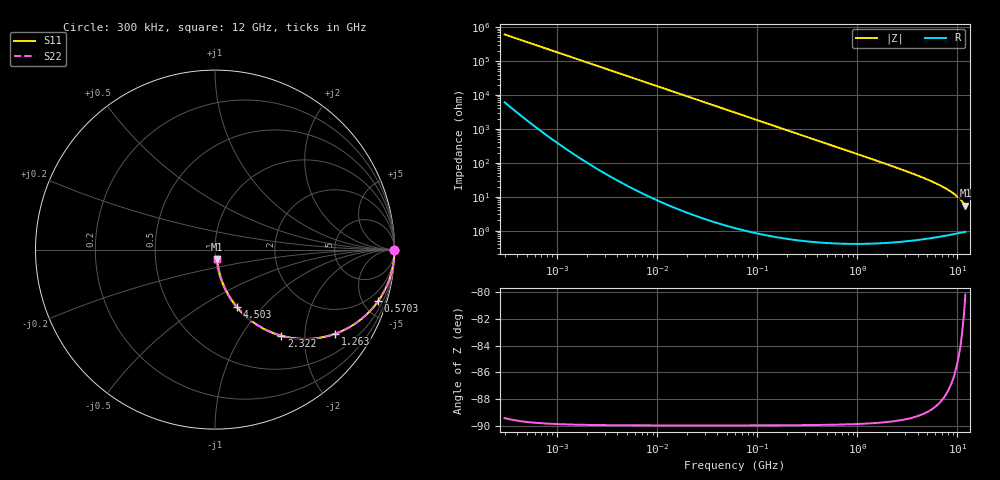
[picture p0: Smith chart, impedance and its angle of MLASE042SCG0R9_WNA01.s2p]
! MLASE042SCG0R9_WNA01  S-PARAMETER MODEL  ( General Type )
! Model Generated by TAIYO YUDEN Corporation (http://www.ty-top.com)
! Version 1.0
! TAIYO YUDEN Control No. 130801
! Copyright(c) 2013 TAIYO YUDEN CO.,LTD. All Rights Reserved.
! Product Description (link to TY-COMPAS)
! https://ds.yuden.co.jp/TYCOMPAS/or/detail?pn=MLASE042SCG0R9AWNA01&u=M
! Products Name : Multilayer Ceramic Capacitors
! Characteristics :
!  Capacitance : 0.9 pF , Rated Voltage : 16V , TCC : CG / C0G
!  Case Size : 0.4 x 0.2 / 0.016 x 0.008 [mm/inch] , Thickness : 0.2 / 0.008 [mm/inch]
!  (Conditions: Temperature = 25 degC , DC Bias Current/Voltage = 0A / 0V)
! External Node Assignments :
!  1  o---| |---o  2
! GND o---------o GND
! Frequency Range : 0.3MHz  -  12000MHz  [ 401 STEP ]
# MHz S RI R 50
! Freq[MHz].  S11 Real  S11 Imag  S21 Real  S21 Imag  S12 Real  S12 Imag  S22 Real  S22 Imag
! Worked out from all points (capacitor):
!   401 points, 300 kHz to 12 GHz, reference 50 ohm
!   read as one part in series: C = 876 fF near 316.3 kHz
!   lowest |Z| = 5.43 ohm at 12 GHz (marker M1)
!   S11 on the Smith chart (normalised r, x): 300 kHz: open; 570.3 MHz: 1.01, -6.36; 1.263 GHz: 1.01, -2.86; 2.322 GHz: 1.01, -1.53; 4.503 GHz: 1.01, -0.73; 12 GHz: 1.02, -0.11
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0.3  1 -0.000165  1.68e-06 0.000165  1.68e-06 0.000165  1 -0.000165
1.769972  1 -0.000974  2.14e-06 0.000974  2.14e-06 0.000974  1 -0.000974
10.44266  1 -0.00575  3.55e-05 0.00575  3.55e-05 0.00575  1 -0.00575
60  0.9989 -0.033  0.0011 0.033  0.0011 0.033  0.9989 -0.033
164.1901  0.9918 -0.0897  0.00815 0.0897  0.00815 0.0897  0.9918 -0.0897
244.3004  0.9821 -0.1321  0.0179 0.1321  0.0179 0.1321  0.9821 -0.1321
353.9943  0.9632 -0.1878  0.0368 0.1878  0.0368 0.1878  0.9632 -0.1878
570.2811  0.9097 -0.2859  0.0903 0.2859  0.0903 0.2859  0.9097 -0.2859
848.5281  0.8195 -0.3837  0.1805 0.3837  0.1805 0.3837  0.8195 -0.3837
1021.415  0.7576 -0.4274  0.2424 0.4274  0.2424 0.4274  0.7576 -0.4274
1262.535  0.6707 -0.4685  0.3293 0.4685  0.3293 0.4685  0.6707 -0.4685
1645.489  0.5431 -0.4962  0.4569 0.4962  0.4569 0.4962  0.5431 -0.4962
2088.533  0.4214 -0.4912  0.5786 0.4912  0.5786 0.4912  0.4214 -0.4912
2321.999  0.369 -0.4796  0.631 0.4796  0.631 0.4796  0.369 -0.4796
3276.641  0.22 -0.4096  0.78 0.4096  0.78 0.4096  0.22 -0.4096
4502.883  0.1223 -0.3201  0.8777 0.3201  0.8777 0.3201  0.1223 -0.3201
6354.153  0.0574 -0.2192  0.9426 0.2192  0.9426 0.2192  0.0574 -0.2192
8281.503  0.0294 -0.1463  0.9706 0.1463  0.9706 0.1463  0.0294 -0.1463
9968.853  0.018 -0.0983  0.982 0.0983  0.982 0.0983  0.018 -0.0983
10793.46  0.0148 -0.0784  0.9852 0.0784  0.9852 0.0784  0.0148 -0.0784
11686.27  0.0125 -0.0589  0.9875 0.0589  0.9875 0.0589  0.0125 -0.0589
12000  0.012 -0.0524  0.988 0.0524  0.988 0.0524  0.012 -0.0524
